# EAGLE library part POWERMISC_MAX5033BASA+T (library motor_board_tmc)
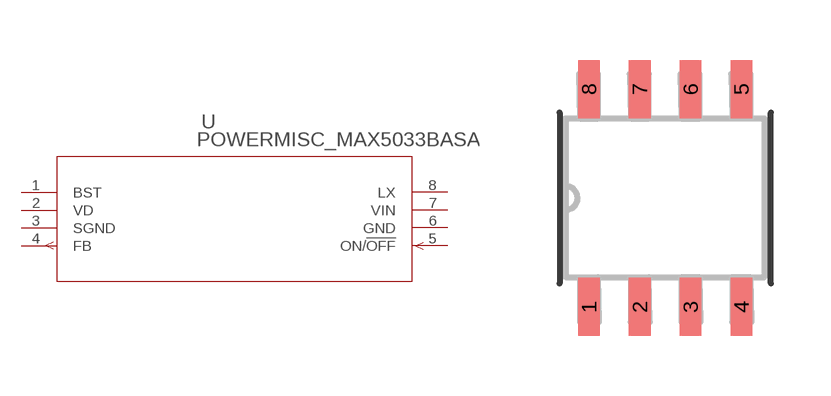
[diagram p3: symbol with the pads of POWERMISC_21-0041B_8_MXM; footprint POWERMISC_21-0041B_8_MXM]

Designator prefix U

## POWERMISC_MAX5033BASA+T (BUILT_BY: EMA_UL_Team; MANUFACTURER_PART_NUMBER: max5033basa+T; SOURCELIBRARY: Maxim_2014-06-20; VENDOR: Maxim Integrated Products)  [POWERMISC_21-0041B_8_MXM]
1  BST  pas
2  VD  pwr
3  SGND  pwr
4  FB  out
5  ON/!OFF  in
6  GND  pwr
7  VIN  pwr
8  LX  pas

## Footprint POWERMISC_21-0041B_8_MXM (pad centres in mm)
smd 0.543 x 1.455: 1 -1.905,-2.721; 2 -0.635,-2.721; 3 0.635,-2.721; 4 1.905,-2.721; 5 1.905,2.721; 6 0.635,2.721; 7 -0.635,2.721; 8 -1.905,2.721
